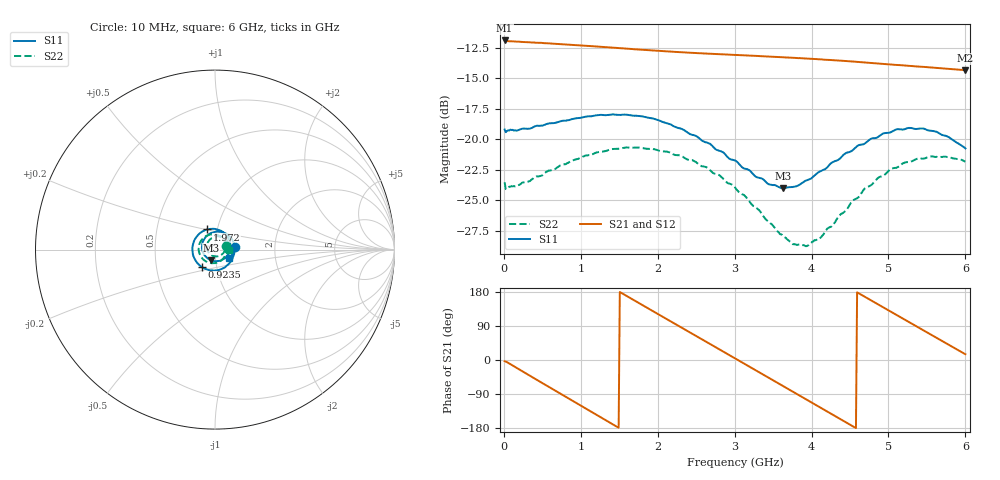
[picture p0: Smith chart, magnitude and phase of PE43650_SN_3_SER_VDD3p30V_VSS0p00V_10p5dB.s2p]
!Keysight Technologies,N5245B,MY57181451,A.13.50.07
!Date: Tuesday, May 07, 2019 08:00:06
!Correction: S11(Full 2 Port(1,2))
!S21(Full 2 Port(1,2))
!S12(Full 2 Port(1,2))
!S22(Full 2 Port(1,2))
!S2P File: Measurements: S11, S21, S12, S22:
# Hz S  dB  R 50
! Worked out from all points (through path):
!   401 points, 10 MHz to 6 GHz, reference 50 ohm
!   highest |S21| = -11.88 dB at 10 MHz (marker M1); lowest = -14.3 dB at 6 GHz (marker M2)
!   group delay of S21, straight-line fit = 325 ps
!   lowest |S11| = -24.0 dB at 3.634 GHz (marker M3), VSWR 1.13, Z = 47.5 - j5.6 ohm
!   |S11| at or under -10 dB: start of sweep to end of sweep
!   |S22| runs from -28.8 to -20.7 dB; largest |S21 - S12| = 0.0023
!   S11 on the Smith chart (normalised r, x): 10 MHz: 1.24, +0.03; 923.5 MHz: 0.85, -0.17; 1.972 GHz: 0.89, +0.20; 6 GHz: 1.16, -0.11
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1e7  -19.20 7.1  -11.88 -3.3  -11.96 -3.3  -23.53 17.2
2.496e8  -19.12 -36.5  -12.01 -30.8  -12.06 -30.8  -23.55 -36.2
5.1915e8  -18.84 -74.2  -12.10 -63.2  -12.15 -63.1  -22.86 -74.6
9.23475e8  -18.29 -126.6  -12.26 -111.5  -12.31 -111.5  -21.68 -124.5
1.013325e9  -18.22 -137.9  -12.30 -122.1  -12.34 -122.1  -21.47 -135.2
1.2679e9  -18.00 -168.1  -12.40 -152.3  -12.46 -152.3  -21.02 -162.9
1.492525e9  -18.00 165.6  -12.50 -178.8  -12.57 -178.8  -20.78 173.3
1.71715e9  -18.06 140.2  -12.61 154.8  -12.67 154.7  -20.68 150.5
1.971725e9  -18.35 112.0  -12.72 125.0  -12.77 125.0  -20.85 125.4
2.01665e9  -18.45 107.0  -12.74 119.7  -12.79 119.7  -20.94 120.9
2.241275e9  -19.02 81.7  -12.83 93.5  -12.88 93.5  -21.30 98.4
2.4659e9  -19.66 55.4  -12.91 67.3  -12.96 67.3  -21.77 76.1
2.750425e9  -20.82 21.8  -13.00 34.0  -13.05 34.1  -22.85 46.5
3.005e9  -21.74 -12.0  -13.07 4.3  -13.13 4.4  -23.96 18.7
3.3045e9  -23.14 -56.2  -13.16 -30.7  -13.21 -30.6  -25.75 -19.6
3.63395e9  -24.03 -110.8  -13.26 -69.3  -13.32 -69.2  -27.94 -70.1
3.7837e9  -23.89 -136.5  -13.31 -86.8  -13.36 -86.7  -28.63 -97.3
4.008325e9  -23.15 -173.0  -13.39 -113.1  -13.45 -113.0  -28.43 -140.4
4.517475e9  -20.98 116.9  -13.61 -172.7  -13.66 -172.6  -25.18 139.3
5.01165e9  -19.46 61.3  -13.84 129.7  -13.90 129.9  -22.54 83.8
5.4609e9  -19.13 16.5  -14.05 77.6  -14.11 77.7  -21.57 41.9
6e9  -20.75 -32.2  -14.33 15.2  -14.37 15.3  -21.85 -2.2
